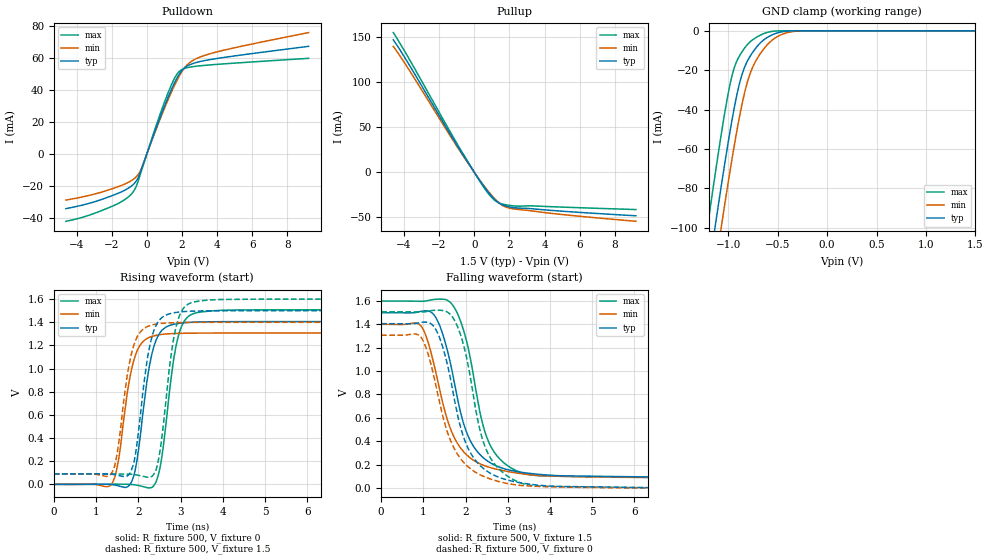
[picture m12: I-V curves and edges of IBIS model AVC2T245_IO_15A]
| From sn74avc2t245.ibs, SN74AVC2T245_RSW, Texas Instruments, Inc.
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[Model]   AVC2T245_IO_15A
Model_type  I/O
Vinl=0.49
Vinh=1.04
Enable   Active-Low
Vref =   0
Rref =   2000
Cref =   15p
Vmeas =   0.75
| variable   typ   min   max
C_comp   5.00pF   4.43pF   5.62pF
| C_pullup   4.73pF   3.29pF   6.96pF
| C_pulldown   4.38pF   4.01pF   4.69pF
| C_tri-state   5.00pF   4.43pF   5.62pF
[Temperature Range]   40   100   -40
| Ambient temperature   25   85   -40
[Voltage range]   1.5   1.4   1.6
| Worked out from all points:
|   slope of the pulldown table from 0 to 0.225 V, typ, clamps not added: 32.1 ohm
|   slope of the pullup table from 0 to 0.225 V, typ, clamps not added: 33.8 ohm
|   GND clamp passes 1 mA (typ) near -0.50 V on its own axis
|   rising waveform, R_fixture 500, V_fixture 0: 20-80 % time 324ps typ, 322ps min, 318ps max; typ from 0 V to 1.41 V
|   falling waveform, R_fixture 500, V_fixture 1.5: 20-80 % time 623ps typ, 667ps min, 558ps max; typ from 1.5 V to 0.09 V
|   rising waveform, R_fixture 500, V_fixture 1.5: 20-80 % time 309ps typ, 310ps min, 304ps max; typ from 0.09 V to 1.5 V
|   falling waveform, R_fixture 500, V_fixture 0: 20-80 % time 626ps typ, 670ps min, 558ps max; typ from 1.41 V to 0 V
[GND Clamp]
| AVC2T245_IO_15A
|   Voltage   I(typ)   I(min)   I(max)
-4.6V     -1.415A    -1.424A    -1.406A
-1.22V    -129.3mA   -150.2mA   -102.9mA
-1.195V   -120.6mA   -141.5mA   -94.12mA
-1.125V   -96.59mA   -117.6mA   -70.08mA
-1.075V   -79.95mA   -100.8mA   -53.65mA
-1.06V    -75.06mA   -95.89mA   -48.92mA
-960mV    -44.57mA   -64.28mA   -22.28mA
-855mV    -21.19mA   -35.79mA   -10.15mA
-745mV    -10.31mA   -17.53mA   -4.232mA
-545mV    -1.808mA   -4.278mA   -210.9uA
-260mV    -2.855uA   -62.75uA   -4.84nA
1.5V      815.1pA    891.9nA    72.11pA
[Pulldown]
| AVC2T245_IO_15A
|   Voltage   I(typ)   I(min)   I(max)
-4.6V     -34.3mA    -28.91mA   -42.24mA
-1.965V   -26.09mA   -21.78mA   -32.79mA
-805mV    -19.46mA   -16.2mA    -24.18mA
-595mV    -16.85mA   -14.27mA   -20.12mA
-345mV    -10.85mA   -10.01mA   -11.9mA
525mV     16.14mA    15.35mA    17.6mA
1.165V    34.37mA    32.9mA     37.17mA
1.61V     45.36mA    43.85mA    48.17mA
1.935V    51.5mA     50.62mA    52.56mA
2.48V     56.15mA    57.63mA    54.52mA
3.355V    58.71mA    62.07mA    55.64mA
9.2V      67.51mA    76.15mA    59.99mA
[Pullup]
| AVC2T245_IO_15A
|   Voltage   I(typ)   I(min)   I(max)
-4.6V     146.8mA    139.5mA    154.8mA
-3.635V   117mA      111.3mA    123.4mA
-1.05V    32.09mA    30.64mA    34.07mA
120mV     -3.581mA   -3.38mA    -3.904mA
745mV     -20.79mA   -19.88mA   -22.2mA
995mV     -26.68mA   -25.76mA   -28.04mA
1.215V    -31.12mA   -30.42mA   -31.92mA
1.44V     -34.55mA   -34.45mA   -34.31mA
1.67V     -36.67mA   -37.47mA   -35.65mA
2.22V     -39.31mA   -40.67mA   -37.34mA
5.31V     -43.72mA   -47.6mA    -38.97mA
9.2V      -48.4mA    -54.5mA    -41.49mA
[Ramp]
| AVC2T245_IO_15A
| variable   typ   min   max
dV/dt_r   0.86/3.36E-10   0.80/3.34E-10   0.92/3.34E-10
dV/dt_f   0.86/6.31E-10   0.79/6.75E-10   0.92/5.69E-10
R_load = 500
[Rising Waveform]
| AVC2T245_IO_15A
R_fixture =   500
C_fixture =   0
L_fixture =   0
V_fixture =   0
V_fixture_min = 0
V_fixture_max = 0
|   Time   V(typ)   V(min)   V(max)
0s        18.53nV    2.897uV    220.4pV
1.36ns    -1.639mV   -380.2uV   1.432mV
1.535ns   -13.22mV   217.7mV    1.499mV
1.8ns     -3.506mV   920.2mV    -74.47uV
1.95ns    169mV      1.133V     -5.993mV
2.35ns    1.166V     1.281V     -17.77mV
2.53ns    1.317V     1.294V     173.8mV
2.955ns   1.39V      1.304V     1.29V
3.48ns    1.403V     1.307V     1.489V
28.38ns   1.406V     1.307V     1.508V
[Falling Waveform]
| AVC2T245_IO_15A
R_fixture =   500
C_fixture =   0
L_fixture =   0
V_fixture =   1.5
V_fixture_min = 1.4
V_fixture_max = 1.6
|   Time   V(typ)   V(min)   V(max)
0s        1.5V       1.4V       1.6V
970ps     1.513V     1.373V     1.597V
1.33ns    1.436V     934.3mV    1.615V
1.675ns   1.012V     477.8mV    1.574V
2.035ns   467.6mV    279.8mV    1.242V
2.36ns    278.4mV    203mV      618.3mV
2.575ns   217.3mV    174.9mV    372.5mV
2.98ns    157.4mV    141.5mV    194.7mV
3.57ns    122mV      111mV      109.5mV
28.38ns   89.98mV    88.21mV    88.17mV
[Rising Waveform]
| AVC2T245_IO_15A
R_fixture =   500
C_fixture =   0
L_fixture =   0
V_fixture =   1.5
V_fixture_min = 1.4
V_fixture_max = 1.6
|   Time   V(typ)   V(min)   V(max)
0s        89.98mV    88.21mV    88.17mV
1.355ns   88.14mV    90.44mV    89.52mV
1.495ns   80.18mV    257.4mV    89.5mV
1.8ns     94.52mV    1.065V     87.57mV
1.935ns   265.4mV    1.242V     82.66mV
2.35ns    1.308V     1.379V     79.23mV
2.505ns   1.42V      1.389V     268.5mV
2.91ns    1.486V     1.397V     1.382V
3.47ns    1.498V     1.399V     1.585V
28.38ns   1.5V       1.4V       1.6V
[Falling Waveform]
| AVC2T245_IO_15A
R_fixture =   500
C_fixture =   0
L_fixture =   0
V_fixture =   0
V_fixture_min = 0
V_fixture_max = 0
|   Time   V(typ)   V(min)   V(max)
0s        1.406V     1.307V     1.508V
970ps     1.418V     1.276V     1.506V
1.325ns   1.336V     830.4mV    1.521V
1.655ns   914.1mV    396.4mV    1.479V
2.01ns    380.9mV    197.7mV    1.141V
2.32ns    201.4mV    117mV      530.7mV
2.515ns   142mV      85.77mV    308.2mV
2.94ns    72.6mV     41.25mV    115.3mV
3.555ns   30.04mV    14.75mV    21.19mV
28.38ns   87.21nV    3.013uV    131.6nV
